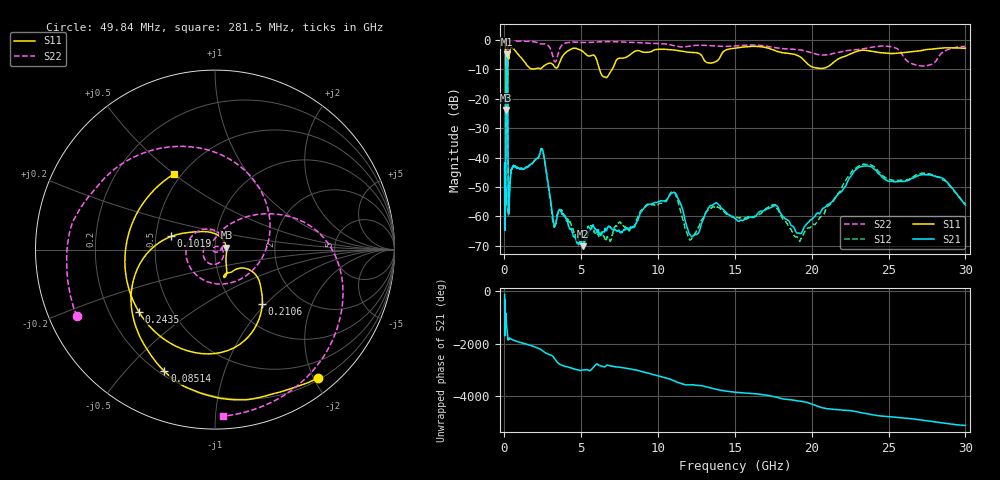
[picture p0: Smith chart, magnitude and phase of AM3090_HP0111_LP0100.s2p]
! Date/Time: Thu, Feb 28, 2019 2:00 PM
! Network Analyzer: Agilent Technologies E8364B Rev: A.07.50.67
! Sweep from 0.010 to 30.000 GHz, 1601 Points, Sweep Type: LOG
! Power Supply: 5.023 V, 0.002 A
# Hz S DB R 50
!freq MagS11 AngS11 MagS21 AngS21 MagS12 AngS12 MagS22 AngS22
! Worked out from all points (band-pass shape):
!   1601 points, 10 MHz to 30 GHz, reference 50 ohm
!   highest |S21| = -4.85 dB at 151.4 MHz (marker M1); lowest = -70.1 dB at 5.128 GHz (marker M2)
!   |S21| within 3 dB of the highest: 112.8 MHz to 197.8 MHz (84.98 MHz wide, 54.7 % of centre)
!   lowest |S11| = -23.8 dB at 109.9 MHz (marker M3), VSWR 1.14, Z = 56.8 + j1.32 ohm
!   |S11| at or under -10 dB: 100.8 MHz to 201.2 MHz (100.5 MHz wide, 66.5 % of centre); 6.184 GHz to 7.008 GHz (824 MHz wide, 12.5 % of centre)
!   |S22| runs from -39.1 to -0.1 dB; largest |S21 - S12| = 0.015
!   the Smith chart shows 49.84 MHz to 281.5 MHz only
!   S11 on the Smith chart (normalised r, x): 49.84 MHz: 0.23, -2.07; 85.14 MHz: 0.22, -0.64; 101.9 MHz: 0.60, +0.10; 210.6 MHz: 1.32, -0.96; 243.5 MHz: 0.33, -0.32; 281.5 MHz: 0.46, +0.50
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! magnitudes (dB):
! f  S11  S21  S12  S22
! 10 MHz  -0.3  -41.7  -43.3  -0.5
! 38.04 MHz  -0.5  -63.4  -58.1  -1.3
! 49.84 MHz  -0.8  -50.0  -48.3  -1.4
! 85.14 MHz  -2.7  -53.2  -52.7  -5.5
! 101.9 MHz  -11.9  -17.1  -17.1  -14.9
! 109.9 MHz  -23.8  -9.1  -9.1  -17.0
! 134.2 MHz  -15.9  -5.2  -5.2  -38.7
! 144.7 MHz  -16.6  -4.9  -4.9  -31.0
! 151.4 MHz  -16.7  -4.9  -4.8  -25.2
! 186.8 MHz  -14.5  -6.1  -6.1  -26.1
! 210.6 MHz  -7.9  -14.0  -14.0  -11.0
! 243.5 MHz  -5.2  -55.2  -57.4  -1.4
! 281.5 MHz  -6.4  -57.6  -57.4  -0.6
! 550.5 MHz  -2.9  -43.0  -43.2  -0.2
! 2.084 GHz  -9.7  -40.4  -40.5  -0.8
! 5.128 GHz  -4.0  -70.1  -68.6  -0.8
! 7.926 GHz  -5.8  -64.1  -64.3  -0.7
! 10.86 GHz  -3.3  -52.2  -51.8  -1.7
! 12.25 GHz  -4.2  -66.7  -67.1  -1.9
! 19.41 GHz  -6.4  -64.8  -66.7  -3.5
! 23.48 GHz  -3.5  -42.9  -42.3  -2.9
! 30 GHz  -2.8  -56.2  -55.9  -2.2
